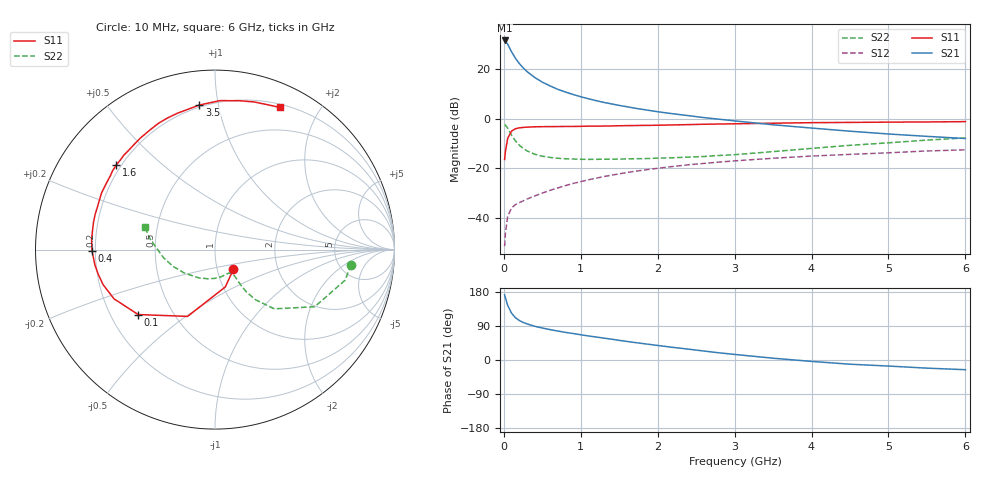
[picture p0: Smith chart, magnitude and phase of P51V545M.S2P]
! SIEMENS Small Signal Semiconductors
! BFP183
! Si NPN RF Bipolar Junction Transistor in SOT143
! VCE = 1.5 V  IC = 45 mA
! Common Emitter S-Parameters:  March  1996
# GHz  S  MA  R  50
!  f  S11  S21  S12  S22
! GHz  MAG  ANG  MAG  ANG  MAG  ANG  MAG  ANG
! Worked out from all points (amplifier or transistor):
!   36 points, 10 MHz to 6 GHz, reference 50 ohm
!   highest |S21| = 31.5 dB at 10 MHz (marker M1)
!   |S21| within 3 dB of that: start of sweep to 74.36 MHz
!   unconditionally stable (mu >= 1): start of sweep to 25.41 MHz; 223.8 MHz to end of sweep
!   at 250 MHz: K = 1.07, MAG = 25.2 dB, |S12| = -33.2 dB
!   at 1.4 GHz: K = 1.65, MAG = 9.6 dB, |S12| = -22.8 dB
!   at 6 GHz: K = 1.30, MAG = -1.0 dB, |S12| = -12.6 dB
!   S11 on the Smith chart (normalised r, x): 10 MHz: 1.20, -0.27; 100 MHz: 0.32, -0.33; 400 MHz: 0.19, -0.01; 1.6 GHz: 0.18, +0.36; 3.5 GHz: 0.19, +0.88; 6 GHz: 0.23, +1.53
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0.01  0.1506 -47.1  37.62 172.1  0.0027 70.0  0.7616 -6.4
0.02  0.2159 -74.6  36.75 164.5  0.0048 73.7  0.745 -13.2
0.05  0.4022 -112.3  31.54 144.2  0.0108 63.0  0.6404 -29.8
0.1  0.5606 -139.8  22.29 123.6  0.0159 48.0  0.4667 -45.0
0.15  0.6258 -154.0  16.57 111.8  0.0185 45.0  0.3582 -51.1
0.2  0.6533 -162.6  12.96 104.4  0.0203 46.1  0.2931 -53.4
0.25  0.6656 -168.4  10.6 99.2  0.022 46.4  0.2529 -53.9
0.3  0.6747 -172.8  8.929 95.4  0.024 48.7  0.2251 -53.9
0.4  0.6852 -179.4  6.785 89.1  0.0277 52.5  0.1926 -53.5
0.5  0.6898 175.4  5.438 84.4  0.0317 54.4  0.1752 -53.6
0.6  0.6908 170.8  4.583 80.2  0.0359 56.9  0.1657 -54.0
0.7  0.6939 167.2  3.903 76.5  0.0402 58.0  0.1594 -54.9
0.9  0.6965 160.2  3.07 69.9  0.0495 59.4  0.1539 -58.3
1.1  0.7064 153.6  2.517 63.4  0.0588 59.4  0.1513 -62.7
1.3  0.7096 148.2  2.125 57.7  0.0681 58.6  0.1523 -68.1
1.6  0.7243 139.5  1.737 49.0  0.0821 57.0  0.1547 -76.8
2.2  0.7478 123.7  1.254 33.3  0.1089 51.5  0.163 -97.6
2.8  0.7798 109.7  0.974 18.9  0.1334 45.3  0.1813 -119.4
3.5  0.8102 96.2  0.753 4.7  0.1593 38.1  0.2169 -143.6
4.5  0.8404 80.8  0.559 -11.1  0.1909 27.5  0.2903 -171.0
5.5  0.8582 70.3  0.44 -21.5  0.2233 18.3  0.3698 170.1
6  0.8709 65.4  0.398 -25.6  0.2357 13.1  0.4092 162.3
